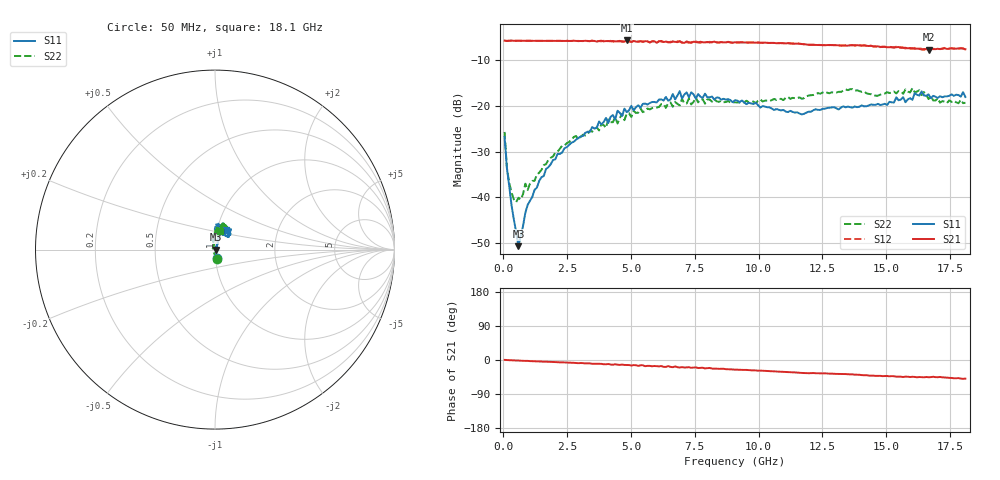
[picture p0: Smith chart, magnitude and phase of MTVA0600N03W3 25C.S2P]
! Network Analyzer HP8720D.06.14 Serial No. US36140669
!  8 Jul 2005  09:51:01
! Frequency  S11  S21  S12  S22
# HZ  S  DB R 50
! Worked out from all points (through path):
!   201 points, 50 MHz to 18.1 GHz, reference 50 ohm
!   highest |S21| = -5.62 dB at 4.833 GHz (marker M1); lowest = -7.6 dB at 16.66 GHz (marker M2)
!   group delay of S21, straight-line fit = 7.74 ps
!   lowest |S11| = -50.8 dB at 591.5 MHz (marker M3), VSWR 1.01, Z = 50.3 - j0.000565 ohm
!   |S11| at or under -10 dB: start of sweep to end of sweep
!   |S22| runs from -41.1 to -16.1 dB; largest |S21 - S12| = 0.019
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5e7  -26.79 -77.1  -5.65 0.3  -5.66 0.3  -25.70 -74.9
1.4025e8  -33.62 -72.6  -5.73 -0.2  -5.71 -0.2  -33.66 -105.4
2.305e8  -37.56 -67.6  -5.68 -0.5  -5.68 -0.5  -36.84 -122.7
4.11e8  -44.88 -52.9  -5.70 -1.1  -5.69 -1.2  -40.51 -154.8
5.915e8  -50.77 -0.1  -5.66 -1.3  -5.70 -1.4  -40.14 174.9
6.8175e8  -48.45 27.9  -5.69 -1.8  -5.70 -1.8  -40.53 163.8
8.6225e8  -43.44 48.1  -5.68 -2.2  -5.70 -2.2  -37.05 153.8
9.525e8  -41.73 54.0  -5.69 -2.4  -5.68 -2.5  -38.45 140.8
1.6745e9  -33.82 62.8  -5.69 -4.5  -5.70 -4.6  -32.77 111.0
3.1185e9  -26.59 72.2  -5.73 -8.2  -5.76 -8.5  -26.31 102.9
4.83325e9  -21.34 79.1  -5.62 -13.0  -5.75 -13.8  -21.69 87.1
6.09675e9  -18.60 76.5  -5.82 -16.8  -5.75 -16.8  -20.22 87.0
6.7285e9  -18.56 83.7  -5.93 -17.0  -6.11 -17.9  -19.12 82.0
6.909e9  -16.74 82.5  -5.76 -20.0  -5.89 -18.9  -19.88 80.3
6.99925e9  -18.38 82.1  -6.05 -18.8  -6.13 -20.3  -18.40 82.0
7.54075e9  -18.40 79.1  -5.97 -19.4  -5.85 -21.4  -18.12 86.1
9.075e9  -18.73 88.2  -6.03 -24.9  -6.01 -25.0  -19.19 77.0
1.21435e10  -20.93 72.3  -6.57 -34.4  -6.53 -34.7  -17.59 73.8
1.512175e10  -19.09 45.5  -7.11 -43.0  -6.97 -42.6  -17.15 74.7
1.602425e10  -18.65 53.0  -7.30 -44.2  -7.44 -46.1  -16.07 68.0
1.6656e10  -17.45 54.4  -7.63 -45.5  -7.56 -44.5  -18.47 63.6
1.81e10  -18.02 61.0  -7.54 -49.1  -7.66 -50.0  -19.30 74.9
